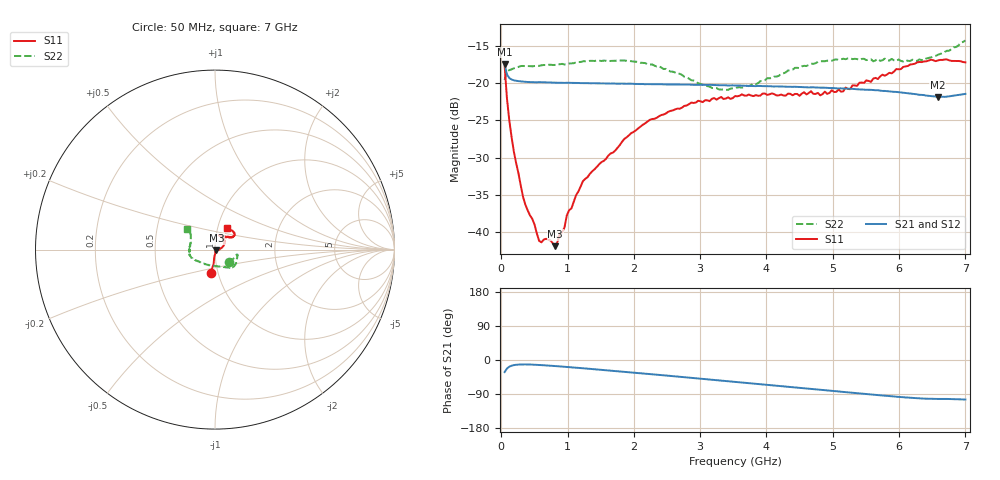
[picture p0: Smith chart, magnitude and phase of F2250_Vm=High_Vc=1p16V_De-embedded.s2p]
! Integrated Device Technology
! Corporate Headquarters
! 6024 Silver Creek Valley Road
! San Jose, CA 95138  USA
! Phone:  1-408-284-8200
! Toll Free:  1-800-223-1366
! Webpage:  http://www.idt.com/
! Timing and RF Division
! 515 Groton Road, Suite 102
! Westford, MA 01886-6024
! Device:  F2250
! Description: Voltage Variable RF Attenuator
! Frequency:  50.0 -  6000.00 MHz
! Package:  3x3 mm Thin QFN Plastic Package: 16 pin
! Ports:  2 RF, 3 DC
!  Pin  1  = GND
!  Pin  2  = NC
!  Pin  3  = RF1  = Port 1
!  Pin  4  = NC
!  Pin  5  = GND
!  Pin  6  = GND
!  Pin  7  = GND
!  Pin  8  = GND
!  Pin  9  = NC
!  Pin 10  = RF2  = Port 2
!  Pin 11  = NC
!  Pin 12  = GND
!  Pin 13  = GND
!  Pin 14  = VCNTRL
!  Pin 15  = VDD
!  Pin 16  = VMODE
! Vcntrl:  1.160 Volts
! Vmode:  +3.300 Volts
! Vdd:  +3.30  Volts
! Current:  1.333 mA
! Data:  The device was measured on a the F2250 evaluation board which has
!  individual transmission lines to the RF pins.  Data was collected
!  using a calibrated network analyzer.  The evaluation board was
!  de-embedded using a TRL calibration technique.
!  The reference plane is the edge of the package pin.
! Misc:  SN 10
!  Action Tracker AT0258
! Date Measured:  2014-11-26
! Date:  2015-10-15  MJV
! Note:
!  Integrated Device Technology supplies this data as a sample of measured
!  data at the package pin for this product.  Your particular data for this
!  product may vary.
!  Data was taken at 25 degrees C.
!  Integrated Device Technology reserves the right to change this data at anytime.
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# GHz S dB R 50
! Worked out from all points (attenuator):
!   201 points, 50 MHz to 7 GHz, reference 50 ohm
!   highest |S21| = -17.47 dB at 50 MHz (marker M1); lowest = -21.9 dB at 6.583 GHz (marker M2)
!   lowest |S11| = -41.9 dB at 814.5 MHz (marker M3), VSWR 1.02, Z = 50.8 - j0.303 ohm
!   |S11| at or under -10 dB: start of sweep to end of sweep
!   |S22| runs from -20.9 to -14.3 dB; largest |S21 - S12| = 0.00041
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0.05  -17.66 -100.8  -17.47 -31.8  -17.48 -31.8  -19.62 -43.3
0.08475  -22.01 -95.4  -18.86 -22.5  -18.86 -22.5  -18.49 -21.6
0.15425  -27.19 -96.0  -19.54 -15.1  -19.53 -15.1  -18.19 -13.3
0.328  -35.26 -84.1  -19.82 -11.6  -19.83 -11.6  -17.72 -12.8
0.50175  -38.98 -68.3  -19.91 -12.4  -19.89 -12.5  -17.73 -16.1
0.57125  -41.17 -53.7  -19.89 -13.1  -19.90 -13.1  -17.71 -17.7
0.6755  -40.88 -48.0  -19.94 -14.3  -19.93 -14.3  -17.61 -19.8
0.8145  -41.87 -21.7  -19.97 -16.0  -19.96 -16.0  -17.58 -23.6
0.884  -40.17 -18.8  -19.98 -16.9  -19.99 -16.9  -17.51 -25.9
0.9535  -39.35 -24.4  -19.99 -17.8  -19.98 -17.8  -17.53 -27.2
0.98825  -37.75 -20.7  -19.98 -18.3  -19.98 -18.3  -17.48 -27.9
1.2315  -33.15 -2.2  -20.02 -21.8  -20.03 -21.8  -17.10 -32.9
1.857  -27.49 17.5  -20.10 -31.2  -20.10 -31.2  -17.00 -42.7
2.37825  -24.47 30.9  -20.17 -39.3  -20.16 -39.3  -17.75 -51.6
3.1775  -22.12 53.4  -20.27 -52.0  -20.26 -52.1  -20.68 -83.7
3.525  -21.76 63.9  -20.34 -57.6  -20.35 -57.6  -20.72 -107.7
4.7065  -21.46 68.2  -20.58 -76.8  -20.59 -76.8  -17.43 -158.6
5.15825  -21.13 51.7  -20.75 -84.1  -20.75 -84.2  -16.76 -167.6
5.85325  -18.64 36.7  -21.13 -95.3  -21.13 -95.4  -17.00 177.0
6.3745  -17.13 38.3  -21.63 -101.9  -21.64 -102.0  -16.95 159.1
6.583  -17.00 42.4  -21.87 -102.8  -21.86 -102.9  -16.24 151.2
7  -17.24 61.9  -21.47 -104.3  -21.46 -104.5  -14.31 144.1
